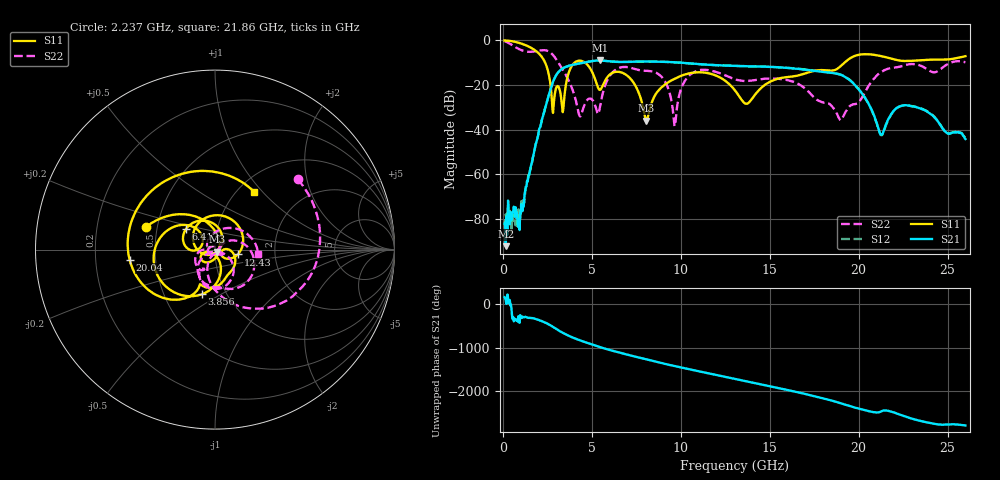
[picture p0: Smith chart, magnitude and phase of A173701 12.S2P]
!  2-Port S-parameters saved by WinCal
! VAR MeasName=S-Parameters (CALIBRATED_DATA) read from VNA (N5245A)
! VAR MeasDate=2017-6-7 10:29:11
! VAR NAME=A173701 12
! VAR FILENAME=A173701 12.S2P
! VAR DATE=2017-6-7 10:29:11
! VAR PHYS_PORTS=1,2
# Hz S DB R 50
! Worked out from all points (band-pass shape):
!   801 points, 100 MHz to 26 GHz, reference 50 ohm
!   highest |S21| = -8.99 dB at 5.442 GHz (marker M1); lowest = -92.3 dB at 164.8 MHz (marker M2)
!   |S21| within 3 dB of the highest: 3.503 GHz to 15.35 GHz (11.84 GHz wide, 126 % of centre)
!   lowest |S11| = -35.9 dB at 8.064 GHz (marker M3), VSWR 1.03, Z = 51.1 - j1.21 ohm
!   |S11| at or under -10 dB: 2.38 GHz to 4.027 GHz (1.646 GHz wide, 51.4 % of centre); 4.624 GHz to 19.2 GHz (14.58 GHz wide, 122 % of centre)
!   |S22| runs from -38.5 to -0.3 dB; largest |S21 - S12| = 0.0044
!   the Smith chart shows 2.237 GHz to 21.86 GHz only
!   S11 on the Smith chart (normalised r, x): 2.237 GHz: 0.44, +0.13; 3.856 GHz: 0.77, -0.41; 6.413 GHz: 0.70, +0.17; 12.43 GHz: 1.29, -0.07; 20.04 GHz: 0.35, -0.05; 21.86 GHz: 1.19, +0.90
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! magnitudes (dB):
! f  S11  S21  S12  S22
! 100 MHz  0.0  -82.3  -89.8  -0.3
! 164.8 MHz  0.0  -92.3  -78.1  -0.5
! 1.039 GHz  -1.4  -73.5  -72.1  -4.3
! 2.237 GHz  -7.9  -34.5  -34.5  -4.4
! 2.852 GHz  -29.6  -17.9  -18.0  -6.8
! 3.856 GHz  -11.7  -11.1  -11.0  -20.8
! 4.438 GHz  -9.2  -10.1  -10.1  -32.6
! 5.442 GHz  -22.2  -9.0  -9.0  -30.6
! 6.413 GHz  -14.1  -9.6  -9.6  -12.8
! 8.064 GHz  -35.9  -9.5  -9.5  -13.6
! 8.744 GHz  -22.5  -9.5  -9.5  -15.1
! 9.651 GHz  -17.2  -9.8  -9.8  -38.5
! 10.52 GHz  -14.7  -10.3  -10.4  -15.4
! 12.43 GHz  -17.7  -11.2  -11.3  -15.4
! 13.05 GHz  -22.4  -11.4  -11.4  -17.4
! 17.39 GHz  -13.8  -13.6  -13.4  -24.7
! 18.97 GHz  -11.6  -15.4  -15.3  -35.8
! 20.04 GHz  -6.4  -22.3  -22.3  -27.4
! 21.24 GHz  -7.0  -42.2  -42.5  -14.3
! 21.69 GHz  -7.9  -34.9  -35.2  -12.6
! 21.86 GHz  -8.2  -32.7  -32.9  -12.4
! 26 GHz  -7.1  -44.2  -44.3  -9.9
